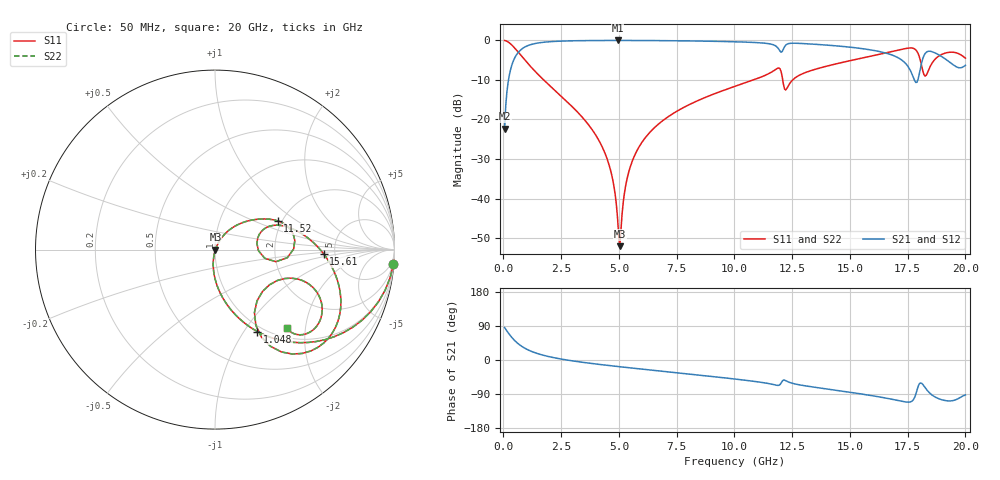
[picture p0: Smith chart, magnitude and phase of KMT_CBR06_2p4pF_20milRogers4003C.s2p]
! Data measured by Modelithics Inc. support@modelithics.com 813-866-6335
! KEMET CBR0603 2.4pF, Pad Width= 0.851mm, Pad Length= 0.64mm, Pad Gap= 0.62mm, 20mil Rogers 4003C substrate Data, January 2022
# hz S ma R 50
! 2 Port Network Data from SP1.SP block
! freq  magS11  angS11  magS21  angS21  magS12  angS12  magS22  angS22
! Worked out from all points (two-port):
!   401 points, 50 MHz to 20 GHz, reference 50 ohm
!   highest |S21| = -0.02 dB at 4.938 GHz (marker M1); lowest = -22.4 dB at 50 MHz (marker M2)
!   |S21| within 3 dB of the highest: 644.1 MHz to 16.43 GHz (15.78 GHz wide, 185 % of centre); 18.3 GHz to 18.63 GHz (323.9 MHz wide, 1.75 % of centre)
!   lowest |S11| = -52.0 dB at 5.037 GHz (marker M3), VSWR 1.01, Z = 50.2 - j0.0405 ohm
!   |S11| at or under -10 dB: 1.742 GHz to 10.82 GHz (9.083 GHz wide, 145 % of centre); 12.09 GHz to 12.52 GHz (431.6 MHz wide, 3.51 % of centre)
!   |S22| runs from -52.0 to 0.0 dB; largest |S21 - S12| = 0
!   S11 on the Smith chart (normalised r, x): 50 MHz: 1, -25; 1.048 GHz: 0.93, -1.15; 11.52 GHz: 1.90, +0.71; 15.61 GHz: 4.04, -0.29; 20 GHz: 1.17, -1.60
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5e7  0.9971 -4.5  0.07619 85.4  0.07619 85.4  0.9971 -4.5
3.99125e8  0.8519 -32.9  0.5226 57.0  0.5226 57.0  0.8519 -32.9
1.0475e9  0.5138 -62.7  0.8566 27.2  0.8566 27.2  0.5138 -62.7
3.391625e9  0.1084 -94.7  0.9919 -5.8  0.9919 -5.8  0.1084 -94.7
4.488875e9  0.03173 -99.8  0.997 -14.1  0.997 -14.1  0.03173 -99.8
4.73825e9  0.01691 -97.6  0.9973 -15.8  0.9973 -15.8  0.01691 -97.6
4.93775e9  0.005793 -82.1  0.9974 -17.1  0.9974 -17.1  0.005793 -82.1
5.0375e9  0.002504 -9.3  0.9973 -17.8  0.9973 -17.8  0.002504 -9.3
5.586125e9  0.03022 63.6  0.9967 -21.4  0.9967 -21.4  0.03022 63.6
6.73325e9  0.08855 59.3  0.9929 -28.8  0.9929 -28.8  0.08855 59.3
1.0025e10  0.2625 38.8  0.9599 -50.2  0.9599 -50.2  0.2625 38.8
1.152125e10  0.3844 24.6  0.9042 -62.6  0.9042 -62.6  0.3844 24.6
1.192025e10  0.4476 6.6  0.7744 -66.7  0.7744 -66.7  0.4476 6.6
1.226938e10  0.2462 15.1  0.8921 -56.0  0.8921 -56.0  0.2462 15.1
1.336662e10  0.4193 17.7  0.8972 -71.0  0.8972 -71.0  0.4193 17.7
1.5611e10  0.6052 -2.2  0.7805 -90.8  0.7805 -90.8  0.6052 -2.2
1.670825e10  0.7099 -15.0  0.6699 -102.2  0.6699 -102.2  0.7099 -15.0
1.785538e10  0.7564 -49.9  0.2933 -89.7  0.2933 -89.7  0.7564 -49.9
1.815462e10  0.4141 -58.0  0.5867 -64.3  0.5867 -64.3  0.4141 -58.0
1.845388e10  0.4528 -20.6  0.7292 -87.2  0.7292 -87.2  0.4528 -20.6
1.895262e10  0.6591 -26.1  0.6291 -104.4  0.6291 -104.4  0.6591 -26.1
2e10  0.5956 -47.6  0.484 -92.3  0.484 -92.3  0.5956 -47.6
